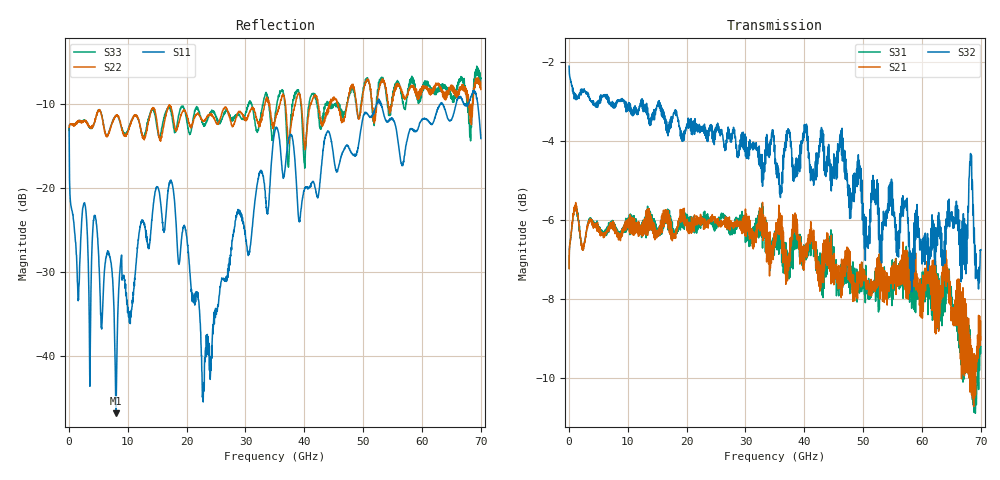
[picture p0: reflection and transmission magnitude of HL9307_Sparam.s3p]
! 2/22/2024 12:45:49 PM
! H:\PRODUCTION_DATA\TEMP_S3P.S3P
! CHANNEL.1
! TR.MEASUREMENT
! CORRECTED.DATA
# GHZ S RI R 50.0
! FREQ.GHZ  S11RE  S11IM  S12RE  S12IM  S13RE  S13IM
!  S21RE  S21IM  S22RE  S22IM  S23RE  S23IM
!  S31RE  S31IM  S32RE  S32IM  S33RE  S33IM
!; PortSelection: Port_123
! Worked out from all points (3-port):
!   2000 points, 35 MHz to 70 GHz, reference 50 ohm
!   strongest paths, dB at 35 MHz, 17.54 GHz, 35.03 GHz, 52.53 GHz, 70 GHz:
!     S32: -2.1, -3.4, -4.6, -5.1, -6.8
!     S21: -7.2, -6.4, -6.3, -7.2, -9.0
!     S31: -7.2, -6.2, -6.7, -7.1, -9.2
!   lowest |S11| = -46.9 dB at 7.98 GHz (marker M1), VSWR 1.01, Z = 50 - j0.453 ohm
!   |S11| at or under -10 dB: start of sweep to 52.3 GHz; 53.1 GHz to 63.12 GHz (10.01 GHz wide, 17.2 % of centre); 63.48 GHz to 65.76 GHz (2.278 GHz wide, 3.52 % of centre)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
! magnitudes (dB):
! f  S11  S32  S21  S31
! 35 MHz  -12.9  -2.1  -7.2  -7.2
! 1.505 GHz  -32.1  -2.9  -5.9  -5.8
! 4.48 GHz  -23.4  -3.1  -6.1  -6.2
! 7.98 GHz  -46.9  -3.1  -6.3  -6.2
! 17.32 GHz  -19.0  -3.7  -6.0  -6.5
! 22.93 GHz  -43.2  -3.7  -6.2  -5.8
! 35.03 GHz  -13.1  -4.6  -6.3  -6.7
! 39.2 GHz  -23.8  -4.8  -6.4  -7.0
! 52.6 GHz  -9.8  -6.3  -7.2  -8.3
! 70 GHz  -14.1  -6.8  -9.0  -9.2
